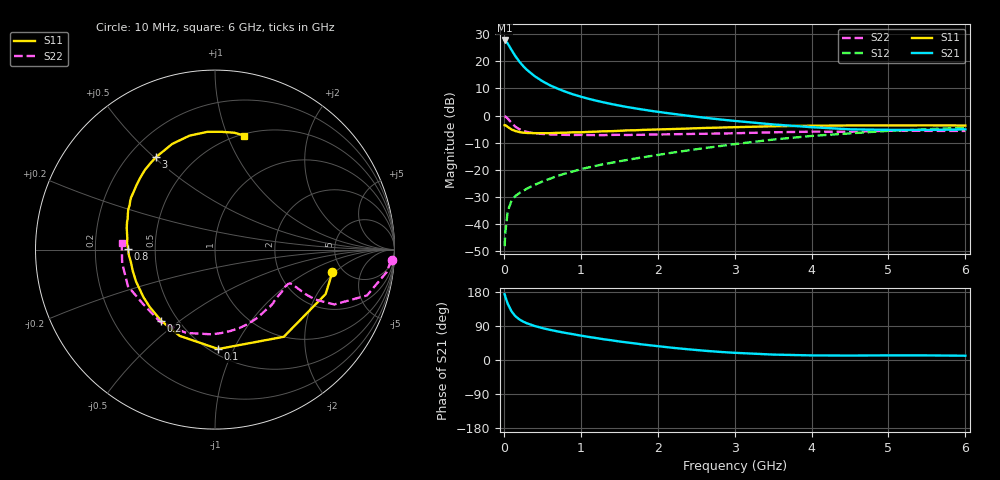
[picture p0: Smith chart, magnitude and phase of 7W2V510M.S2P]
! Infineon Technologies  Discrete & RF Semiconductors
! BFS17W
! Si NPN RF Bipolar Junction Transistor in SOT323
! VCE = 2.5 V  IC = 10 mA
! Common Emitter S-Parameters:  August  1999
# GHz  S  MA  R  50
!  f  S11  S21  S12  S22
! GHz  MAG  ANG  MAG  ANG  MAG  ANG  MAG  ANG
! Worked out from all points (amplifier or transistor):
!   36 points, 10 MHz to 6 GHz, reference 50 ohm
!   highest |S21| = 27.7 dB at 10 MHz (marker M1)
!   |S21| within 3 dB of that: start of sweep to 89.27 MHz
!   unconditionally stable (mu >= 1): 386.3 MHz to 2.724 GHz; 4.249 GHz to end of sweep
!   at 250 MHz: K = 0.81, MSG = 23.1 dB, |S12| = -27.8 dB
!   at 1.4 GHz: K = 1.23, MAG = 8.0 dB, |S12| = -17.4 dB
!   at 6 GHz: K = 1.08, MAG = -2.0 dB, |S12| = -4.5 dB
!   S11 on the Smith chart (normalised r, x): 10 MHz: 4.09, -1.87; 100 MHz: 0.55, -0.87; 200 MHz: 0.41, -0.43; 800 MHz: 0.35, +0.01; 3 GHz: 0.31, +0.51; 6 GHz: 0.52, +1.15
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0.01  0.6659 -11.0  24.33 173.7  0.0039 85.3  0.9853 -3.4
0.02  0.6643 -21.9  23.84 166.6  0.0071 81.8  0.9632 -7.6
0.05  0.6188 -51.7  21.37 148.7  0.0171 69.4  0.8844 -16.8
0.1  0.5542 -88.1  16.24 128.4  0.027 57.9  0.7313 -24.7
0.15  0.5195 -112.3  12.49 115.5  0.0329 53.1  0.6232 -26.5
0.2  0.4972 -127.3  9.976 107.5  0.0371 53.1  0.5625 -26.2
0.25  0.4844 -138.5  8.229 101.5  0.0407 52.8  0.5227 -25.4
0.3  0.4787 -146.3  6.981 96.9  0.0449 54.2  0.5004 -24.9
0.4  0.4745 -158.0  5.349 89.8  0.0527 57.0  0.4714 -24.2
0.5  0.4733 -165.6  4.324 84.3  0.0607 59.4  0.4587 -24.2
0.6  0.4737 -171.4  3.621 79.6  0.0684 61.1  0.4506 -25.1
0.8  0.4839 179.3  2.762 71.5  0.0855 63.5  0.441 -28.3
0.9  0.4914 175.9  2.465 68.0  0.0933 64.0  0.4385 -30.2
1.1  0.4995 169.0  2.045 61.0  0.1106 64.9  0.4379 -34.8
1.3  0.5135 162.7  1.751 54.7  0.1273 65.3  0.4366 -40.0
1.6  0.533 155.1  1.441 46.3  0.1518 65.9  0.4389 -48.2
2.2  0.5654 140.8  1.077 32.1  0.2078 66.3  0.4534 -66.6
3  0.6112 122.4  0.798 19.0  0.2978 62.7  0.4724 -92.2
3.5  0.6354 112.0  0.687 14.3  0.361 58.4  0.4912 -109.1
4.5  0.6574 93.7  0.558 11.7  0.4698 45.9  0.5027 -143.0
5.5  0.66 80.6  0.542 12.1  0.5605 33.5  0.5228 -171.7
6  0.6557 75.5  0.557 11.3  0.5966 27.6  0.521 175.7
